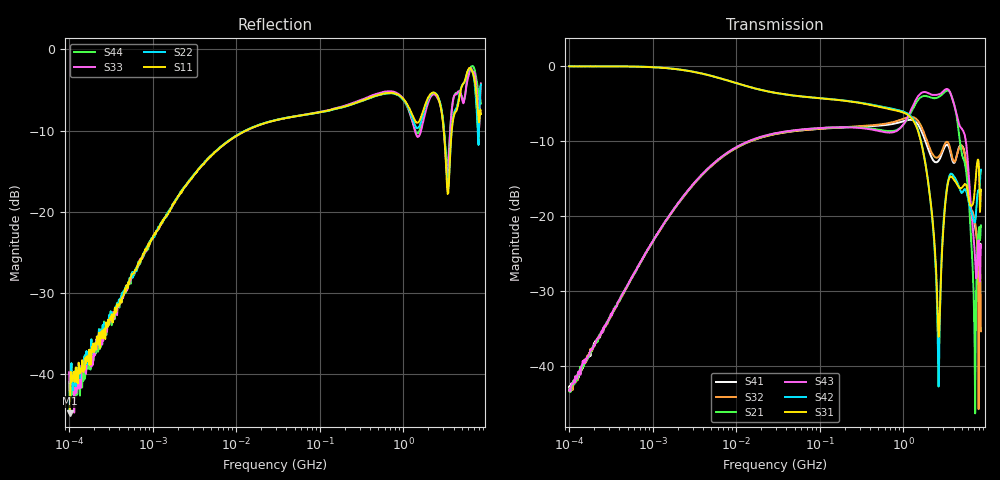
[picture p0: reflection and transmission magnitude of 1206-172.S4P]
!Agilent Technologies,E5071C,MY46110495,A.10.06
!Date: Tue Jun 06 11:21:36 2017
!Data & Calibration Information:
!Freq	S11:SOLT4(ON)	S12:SOLT4(ON)	S13:SOLT4(ON)	S14:SOLT4(ON)
!	S21:SOLT4(ON)	S22:SOLT4(ON)	S23:SOLT4(ON)	S24:SOLT4(ON)
!	S31:SOLT4(ON)	S32:SOLT4(ON)	S33:SOLT4(ON)	S34:SOLT4(ON)
!	S41:SOLT4(ON)	S42:SOLT4(ON)	S43:SOLT4(ON)	S44:SOLT4(ON)
!PortZ  Port1:50+j0  Port2:50+j0  Port3:50+j0  Port4:50+j0
!Above PortZ is port z conversion or system Z0 setting when saving the data.
!When reading, reference impedance value at option line is always used.
# Hz S dB R 50
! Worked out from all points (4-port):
!   801 points, 100 kHz to 8.5 GHz, reference 50 ohm
!   strongest paths, dB at 100 kHz, 1.721 MHz, 29.51 MHz, 502.3 MHz, 8.5 GHz:
!     S31: -0.1, -0.4, -3.6, -5.4, -16.5
!     S42: -0.1, -0.4, -3.6, -5.3, -13.8
!     S43: -43.2, -19.3, -9.0, -8.7, -23.9
!     S21: -43.0, -19.3, -9.0, -8.5, -21.2
!     S32: -43.3, -19.4, -9.1, -7.8, -35.3
!     S41: -42.7, -19.4, -9.1, -8.0, -24.2
!   lowest |S11| = -44.8 dB at 101.7 kHz (marker M1), VSWR 1.01, Z = 50.4 + j0.379 ohm
!   |S11| at or under -10 dB: start of sweep to 13.15 MHz; 3.057 GHz to 3.807 GHz (749.5 MHz wide, 21.8 % of centre)
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100000  -44.58 69.3  -42.97 86.5  -0.06 -0.2  -43.08 -92.7
        -42.98 86.2  -43.02 51.9  -42.90 -93.5  -0.08 -0.2
        -0.07 -0.2  -43.28 -91.0  -39.76 84.7  -42.97 88.5
        -42.75 -91.9  -0.05 -0.3  -43.17 88.8  -40.92 68.2
101665  -44.81 40.9  -43.51 94.1  -0.07 -0.3  -42.73 -88.3
        -43.42 87.0  -44.41 47.0  -43.13 -92.1  -0.08 -0.3
        -0.08 -0.2  -42.88 -87.9  -42.10 88.1  -42.96 89.9
        -42.58 -90.0  -0.06 -0.4  -43.00 87.0  -43.50 67.3
2.909522e7  -8.74 18.4  -9.00 15.6  -3.58 -10.3  -9.09 -166.4
            -9.01 15.5  -8.72 18.2  -9.10 -166.3  -3.60 -10.2
            -3.59 -10.3  -9.10 -166.4  -8.74 18.3  -9.01 15.5
            -9.08 -166.5  -3.59 -10.2  -8.99 15.6  -8.73 18.1
1.295951e9  -8.16 34.7  -5.78 19.4  -7.16 -74.9  -7.23 94.5
            -5.78 19.5  -8.59 32.7  -6.83 93.5  -7.01 -73.6
            -7.18 -74.8  -6.84 93.5  -8.97 24.9  -5.43 23.0
            -7.22 94.5  -6.99 -73.5  -5.42 23.0  -9.00 30.6
2.64856e9  -6.09 87.0  -4.15 -10.3  -36.26 139.0  -12.64 51.1
           -4.16 -10.3  -6.03 89.2  -12.11 45.1  -42.38 136.7
           -36.06 139.8  -12.11 45.2  -6.25 90.3  -3.83 -9.4
           -12.63 51.1  -42.67 137.8  -3.82 -9.5  -6.09 92.4
5.086878e9  -4.41 -76.3  -11.93 -70.0  -16.16 154.6  -10.69 -22.3
            -11.94 -69.9  -4.39 -77.7  -10.79 -28.5  -16.88 158.3
            -16.17 154.6  -10.78 -28.4  -6.22 -90.8  -8.49 -58.8
            -10.68 -22.1  -16.84 158.3  -8.49 -58.7  -5.91 -85.7
8.5e9  -7.96 120.4  -21.15 36.9  -16.44 30.0  -24.20 18.4
       -21.24 37.0  -4.34 130.7  -35.33 -94.4  -13.86 26.4
       -16.49 30.0  -35.32 -94.7  -4.20 133.9  -23.91 19.8
       -24.17 19.2  -13.83 26.7  -23.88 19.9  -6.66 110.2
